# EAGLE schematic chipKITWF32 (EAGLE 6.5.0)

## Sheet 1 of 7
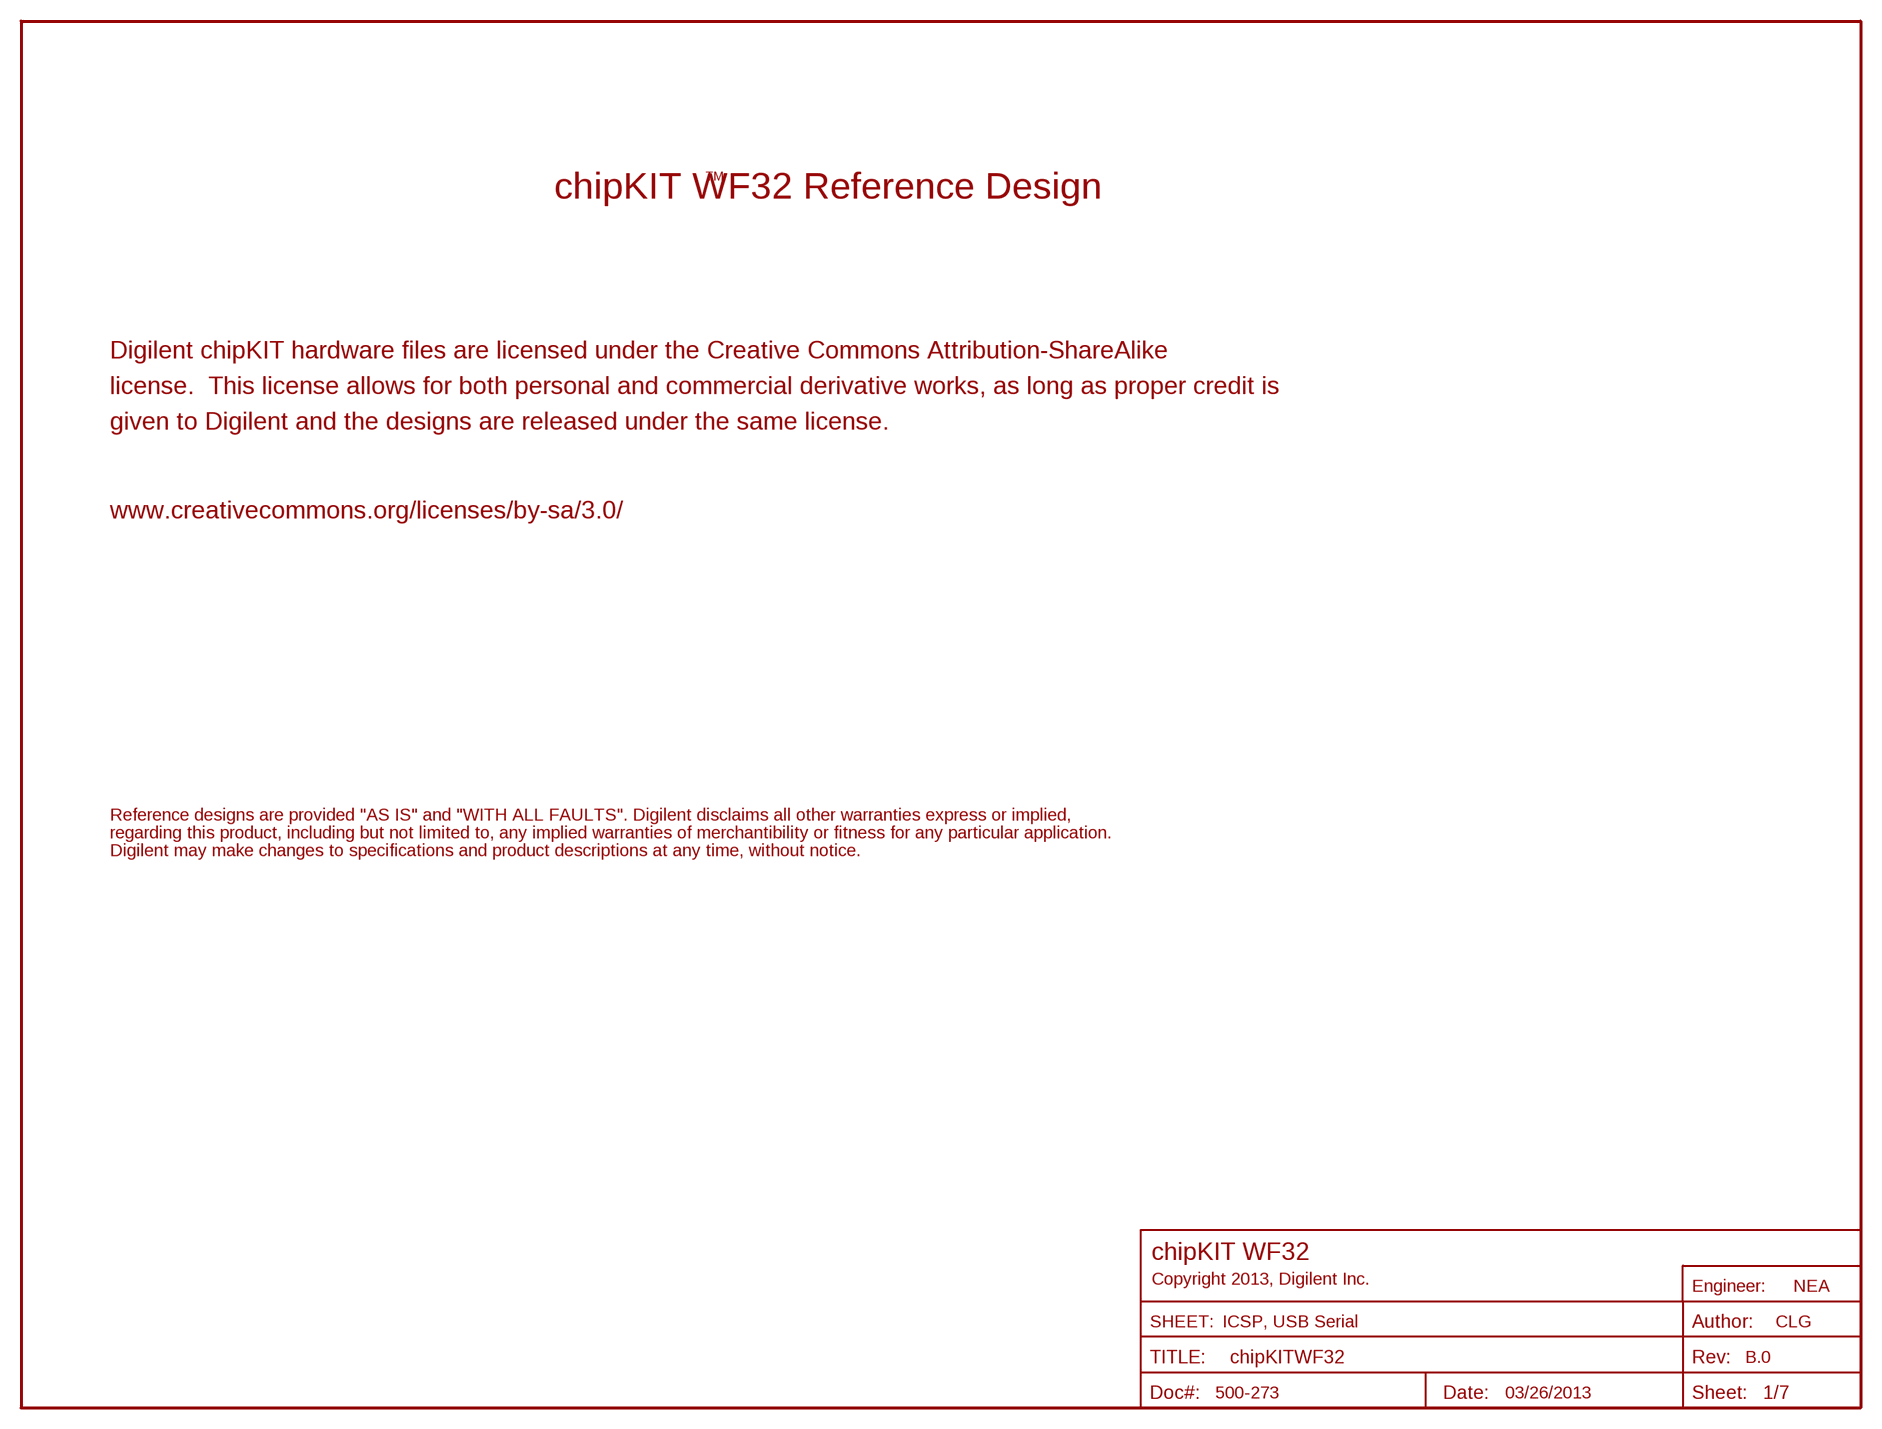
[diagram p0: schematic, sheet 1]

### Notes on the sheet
- TM
- chipKIT WF32 Reference Design
- Digilent chipKIT hardware files are licensed under the Creative Commons Attribution-ShareAlike
- license.  This license allows for both personal and commercial derivative works, as long as proper credit is
- given to Digilent and the designs are released under the same license.
- www.creativecommons.org/licenses/by-sa/3.0/
- Reference designs are provided "AS IS" and "WITH ALL FAULTS". Digilent disclaims all other warranties express or implied,
- regarding this product, including but not limited to, any implied warranties of merchantibility or fitness for any particular application.
- Digilent may make changes to specifications and product descriptions at any time, without notice.
- chipKIT WF32
- Copyright 2013, Digilent Inc.
- NEA
- ICSP, USB Serial | CLG
- B.0
- 500-273 | 03/26/2013

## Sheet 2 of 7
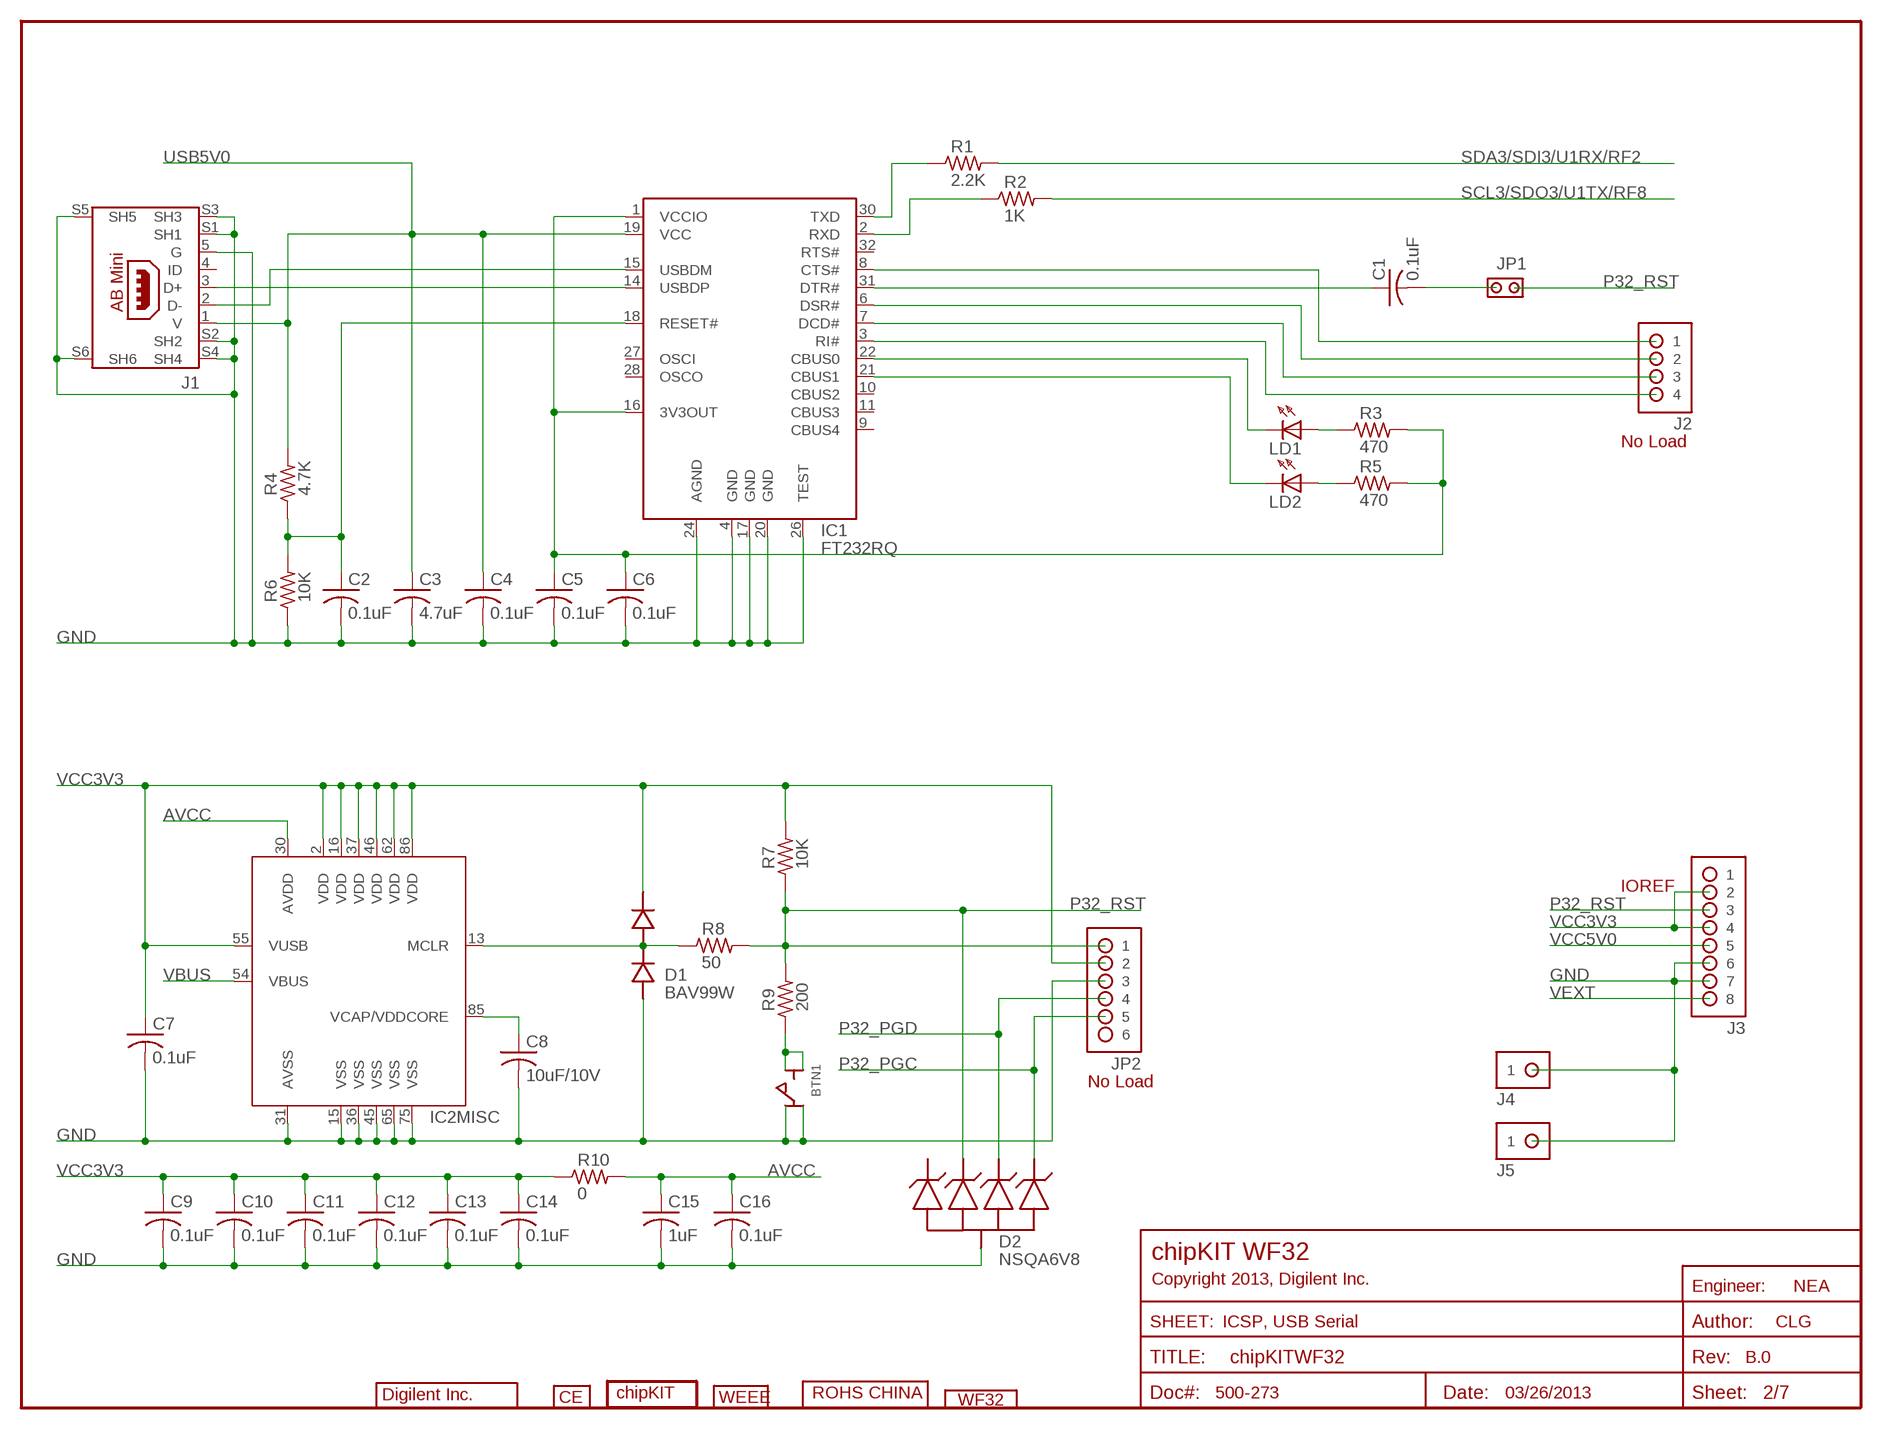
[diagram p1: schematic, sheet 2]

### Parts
BTN1  SW-P8008  [SW-P8008]
C1  0.1uF  CAP-S0402S  [C0402S]
C2  0.1uF  CAP-S0402S  [C0402S]
C3  4.7uF  CAP-S0603S  [C0603S]
C4  0.1uF  CAP-S0402S  [C0402S]
C5  0.1uF  CAP-S0402S  [C0402S]
C6  0.1uF  CAP-S0402S  [C0402S]
C7  0.1uF  CAP-S0402S  [C0402S]
C8  10uF/10V  CAP-S0805S  [C0805S]
C9  0.1uF  CAP-S0402S  [C0402S]
C10  0.1uF  CAP-S0402S  [C0402S]
C11  0.1uF  CAP-S0402S  [C0402S]
C12  0.1uF  CAP-S0402S  [C0402S]
C13  0.1uF  CAP-S0402S  [C0402S]
C14  0.1uF  CAP-S0402S  [C0402S]
C15  1uF  CAP-S0402S  [C0402S]
C16  0.1uF  CAP-S0402S  [C0402S]
D1  BAV99W  [SOT-323]
D2  NSQA6V8  [SOT-323-5]
IC1  FT232RQ  [QFN32]
IC2  PIC32MX695F512L-80I/PT  PIC32MX7X5FL-PT  [TQ100-PT]
J1  USB-AB-MINI  [USB-AB-MINI]
J2  No Load  HDR-1X4  [HDR-1X4]
J3  ST. Female  HDR-1X8  [HDR-1X8]
J4  ST. Male  HDR-1X1  [HDR-1X1]
J5  ST. Male  HDR-1X1  [HDR-1X1]
JP1  ST. Male  JPR-1X2  [JPR-1X2]
JP2  No Load  HDR-1X6-OFFSET  [HDR-1X6_OFFSET]
LD1  Red  LED-S0603S  [D0603S]
LD2  Red  LED-S0603S  [D0603S]
LOGO1  DIGILENT_INC-BT-1000  [DIGILENT_BEYOND_1000_LOGO]
LOGO2  CE  [CE_LOGO]
LOGO3  CHIPKIT  [CHIPKIT_LOGO]
LOGO4  WEEE-S  [WEEE_LOGO]
LOGO5  ROHS-CHINA  [ROHS_CHINA_LOGO]
R1  2.2K  RES-S0402S  [R0402S]
R2  1K  RES-S0402S  [R0402S]
R3  470  RES-S0402S  [R0402S]
R4  4.7K  RES-S0402S  [R0402S]
R5  470  RES-S0402S  [R0402S]
R6  10K  RES-S0402S  [R0402S]
R7  10K  RES-S0402S  [R0402S]
R8  50  RES-S0402S  [R0402S]
R9  200  RES-S0402S  [R0402S]
R10  0  RES-S0603S  [R0603S]
U$1  CHIPKIT_WF32_LOGO  [CHIPKIT_WF32_LOGO]

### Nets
AVCC: C15.1 C16.1 IC2.30(MISC:AVDD) R10.2
FT3V3: C5.1 C6.1 IC1.1(VCCIO) IC1.16(3V3OUT) R3.2 R5.2
GND: BTN1.1A BTN1.2A C2.2 C3.2 C4.2 C5.2 C6.2 C7.2 C8.2 C9.2 C10.2 C11.2 C12.2 C13.2 C14.2 C15.2 C16.2 D1.1(CAT) D2.2(COM) IC1.4(GND) IC1.17(GND) IC1.20(GND) IC1.24(AGND) IC1.26(TEST) IC2.15(MISC:VSS) IC2.31(MISC:AVSS) IC2.36(MISC:VSS) IC2.45(MISC:VSS) IC2.65(MISC:VSS) IC2.75(MISC:VSS) J1.5(G) J1.S1(SH1) J1.S2(SH2) J1.S3(SH3) J1.S4(SH4) J1.S5(SH5) J1.S6(SH6) J3.6 J3.7 J4.1 J5.1 JP2.3 R6.1 ; also sheet 3,4,5,6,7
N$14: C1.2 JP1.2
N$21: D1.3(COM) IC2.13(MISC:MCLR) R8.1
N$24: C8.1 IC2.85(MISC:VCAP/VDDCORE)
N$27: BTN1.1B BTN1.2B R9.1
N$33: IC1.15(USBDM) J1.2(D-)
N$37: IC1.14(USBDP) J1.3(D+)
N$41: IC1.30(TXD) R1.1
N$43: IC1.2(RXD) R2.1
N$47: C2.1 IC1.18(RESET#) R4.1 R6.2
N$52: IC1.8(CTS#) J2.1
N$53: C1.1 IC1.31(DTR#)
N$54: IC1.6(DSR#) J2.2
N$55: IC1.7(DCD#) J2.3
N$56: IC1.3(RI#) J2.4
N$57: IC1.22(CBUS0) LD1.C
N$58: IC1.21(CBUS1) LD2.C
N$59: LD1.A R3.1
N$60: LD2.A R5.1
P32_PGC: D2.5(D4) JP2.5 ; also sheet 4
P32_PGD: D2.4(D3) JP2.4 ; also sheet 4
P32_RST: D2.3(D2) J3.3 JP1.1 JP2.1 R7.1 R8.2 R9.2
SCL3/SDO3/U1TX/RF8: R2.2 ; also sheet 3,5
SDA3/SDI3/U1RX/RF2: R1.2 ; also sheet 3,5
USB5V0: C3.1 C4.1 IC1.19(VCC) J1.1(V) R4.2 ; also sheet 7
VBUS: IC2.54(MISC:VBUS) ; also sheet 6,7
VCC3V3: C7.1 C9.1 C10.1 C11.1 C12.1 C13.1 C14.1 D1.2(AN) IC2.2(MISC:VDD) IC2.16(MISC:VDD) IC2.37(MISC:VDD) IC2.46(MISC:VDD) IC2.55(MISC:VUSB) IC2.62(MISC:VDD) IC2.86(MISC:VDD) J3.2 J3.4 JP2.2 R7.2 R10.1 ; also sheet 4,6,7
VCC5V0: J3.5 ; also sheet 6,7
VEXT: J3.8 ; also sheet 7
Unconnected: D2.1(D1) IC1.9(CBUS4) IC1.10(CBUS2) IC1.11(CBUS3) IC1.27(OSCI) IC1.28(OSCO) IC1.32(RTS#) J1.4(ID) J3.1 JP2.6

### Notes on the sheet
- No Load
- IOREF
- No Load
- chipKIT WF32
- Copyright 2013, Digilent Inc.
- NEA
- ICSP, USB Serial | CLG
- B.0
- 500-273 | 03/26/2013

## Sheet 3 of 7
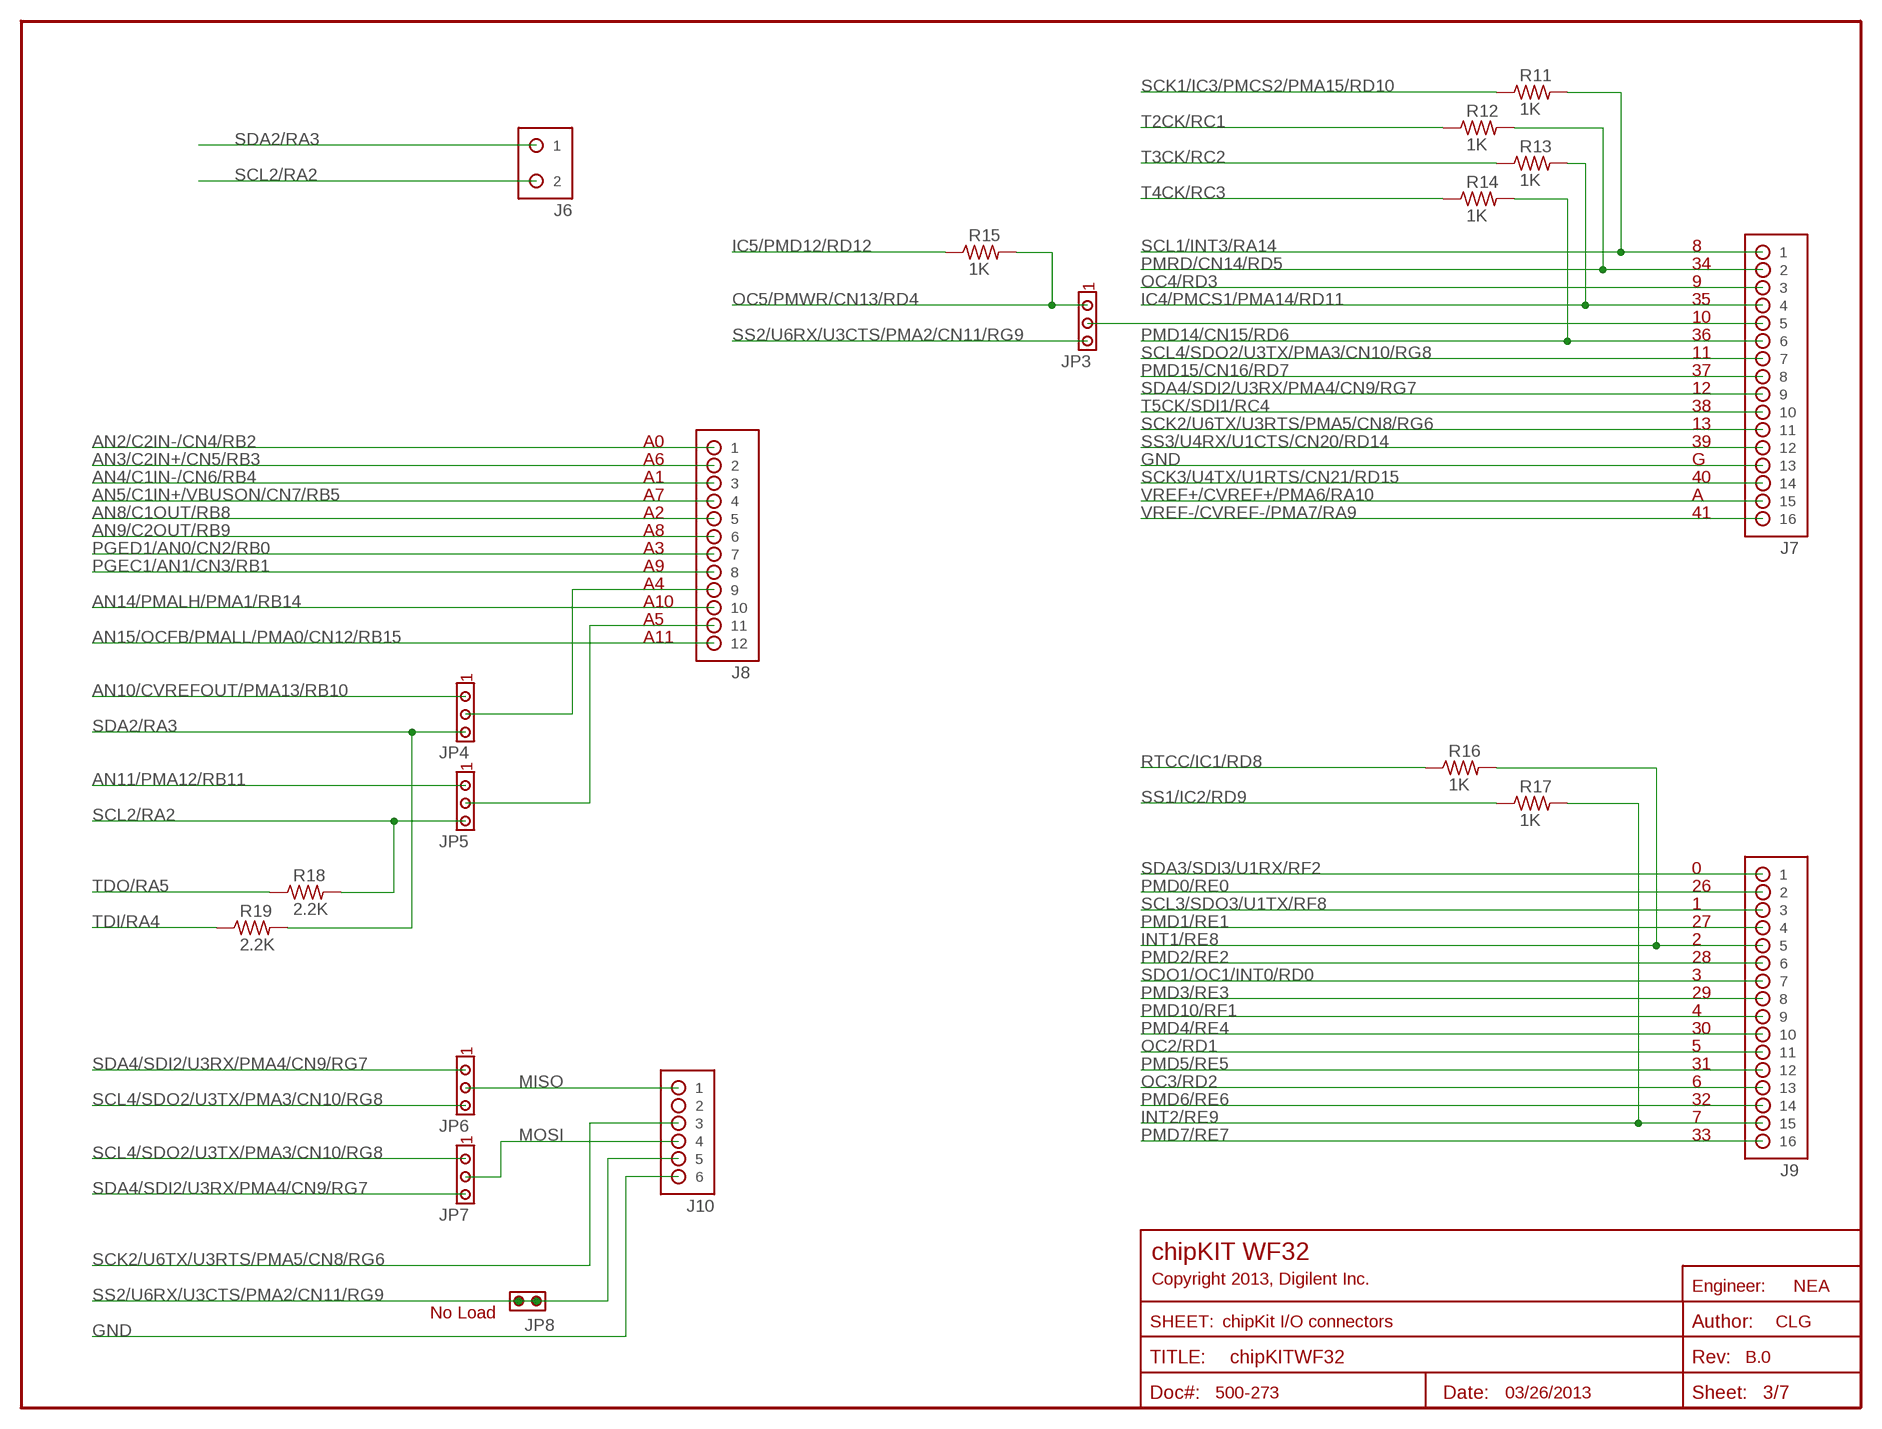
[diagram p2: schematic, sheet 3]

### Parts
J6  ST. Female  HDR-1X2  [HDR-1X2]
J7  ST. Female  HDR-2X8  [HDR-2X8]
J8  ST. Female  HDR-2X6  [HDR-2X6]
J9  ST. Female  HDR-2X8  [HDR-2X8]
J10  ST. Male  HDR-2X3  [HDR-2X3]
JP3  JPR-1X3  [JPR-1X3]
JP4  ST. Male  JPR-1X3  [JPR-1X3]
JP5  ST. Male  JPR-1X3  [JPR-1X3]
JP6  JPR-1X3  [JPR-1X3]
JP7  JPR-1X3  [JPR-1X3]
JP8  No Load  JPR-1X2  [JPR-1X2]
R11  1K  RES-S0402S  [R0402S]
R12  1K  RES-S0402S  [R0402S]
R13  1K  RES-S0402S  [R0402S]
R14  1K  RES-S0402S  [R0402S]
R15  1K  RES-S0402S  [R0402S]
R16  1K  RES-S0402S  [R0402S]
R17  1K  RES-S0402S  [R0402S]
R18  2.2K  RES-S0402S  [R0402S]
R19  2.2K  RES-S0402S  [R0402S]

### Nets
AN2/C2IN-/CN4/RB2: J8.1 ; also sheet 4
AN3/C2IN+/CN5/RB3: J8.2 ; also sheet 4
AN4/C1IN-/CN6/RB4: J8.3 ; also sheet 4
AN5/C1IN+/VBUSON/CN7/RB5: J8.4 ; also sheet 4,6
AN8/C1OUT/RB8: J8.5 ; also sheet 4
AN9/C2OUT/RB9: J8.6 ; also sheet 4
AN10/CVREFOUT/PMA13/RB10: JP4.1 ; also sheet 4
AN11/PMA12/RB11: JP5.1 ; also sheet 4
AN14/PMALH/PMA1/RB14: J8.10 ; also sheet 4
AN15/OCFB/PMALL/PMA0/CN12/RB15: J8.12 ; also sheet 4
GND: J7.13 J10.6 ; also sheet 2,4,5,6,7
IC4/PMCS1/PMA14/RD11: J7.4 R13.2 ; also sheet 5
IC5/PMD12/RD12: R15.1 ; also sheet 5
INT1/RE8: J9.5 R16.2 ; also sheet 5
INT2/RE9: J9.15 R17.2 ; also sheet 5
MISO: J10.1 JP6.2
MOSI: J10.4 JP7.2
N$46: J8.9 JP4.2
N$49: J8.11 JP5.2
N$50: J7.5 JP3.2
OC2/RD1: J9.11 ; also sheet 5
OC3/RD2: J9.13 ; also sheet 5
OC4/RD3: J7.3 ; also sheet 5
OC5/PMWR/CN13/RD4: JP3.1 R15.2 ; also sheet 5
PGEC1/AN1/CN3/RB1: J8.8 ; also sheet 4
PGED1/AN0/CN2/RB0: J8.7 ; also sheet 4
PMD0/RE0: J9.2 ; also sheet 5
PMD1/RE1: J9.4 ; also sheet 5
PMD2/RE2: J9.6 ; also sheet 5
PMD3/RE3: J9.8 ; also sheet 5
PMD4/RE4: J9.10 ; also sheet 5
PMD5/RE5: J9.12 ; also sheet 5
PMD6/RE6: J9.14 ; also sheet 5
PMD7/RE7: J9.16 ; also sheet 5
PMD10/RF1: J9.9 ; also sheet 5
PMD14/CN15/RD6: J7.6 R14.2 ; also sheet 5
PMD15/CN16/RD7: J7.8 ; also sheet 5
PMRD/CN14/RD5: J7.2 R12.2 ; also sheet 5
RTCC/IC1/RD8: R16.1 ; also sheet 5
SCK1/IC3/PMCS2/PMA15/RD10: R11.1 ; also sheet 5
SCK2/U6TX/U3RTS/PMA5/CN8/RG6: J7.11 J10.3 ; also sheet 5,6
SCK3/U4TX/U1RTS/CN21/RD15: J7.14 ; also sheet 5
SCL1/INT3/RA14: J7.1 R11.2 ; also sheet 4,6
SCL2/RA2: J6.2 JP5.3 R18.2 ; also sheet 4
SCL3/SDO3/U1TX/RF8: J9.3 ; also sheet 2,5
SCL4/SDO2/U3TX/PMA3/CN10/RG8: J7.7 JP6.3 JP7.1 ; also sheet 5
SDA2/RA3: J6.1 JP4.3 R19.2 ; also sheet 4
SDA3/SDI3/U1RX/RF2: J9.1 ; also sheet 2,5
SDA4/SDI2/U3RX/PMA4/CN9/RG7: J7.9 JP6.1 JP7.3 ; also sheet 5
SDO1/OC1/INT0/RD0: J9.7 ; also sheet 5
SS1/IC2/RD9: R17.1 ; also sheet 5
SS2/U6RX/U3CTS/PMA2/CN11/RG9: J10.5 JP3.3 JP8.1 JP8.2 ; also sheet 5
SS3/U4RX/U1CTS/CN20/RD14: J7.12 ; also sheet 5
T2CK/RC1: R12.1 ; also sheet 5
T3CK/RC2: R13.1 ; also sheet 5
T4CK/RC3: R14.1 ; also sheet 5
T5CK/SDI1/RC4: J7.10 ; also sheet 5
TDI/RA4: R19.1 ; also sheet 4
TDO/RA5: R18.1 ; also sheet 4
VREF+/CVREF+/PMA6/RA10: J7.15 ; also sheet 4
VREF-/CVREF-/PMA7/RA9: J7.16 ; also sheet 4
Unconnected: J10.2

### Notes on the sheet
- 8
- 34
- 9
- 35
- 10
- 36
- 11
- 37
- 12
- 38
- 13
- A0 | 39
- A6 | G
- A1 | 40
- A7 | A
- A2 | 41
- A8
- A3
- A9
- A4
- A10
- A5
- A11
- 0
- 26
- 1
- 27
- 2
- 28
- 3
- 29
- 4
- 30
- 5
- 31
- 6
- 32
- 7
- 33
- chipKIT WF32
- Copyright 2013, Digilent Inc.
- NEA
- No Load
- chipKit I/O connectors | CLG
- B.0
- 500-273 | 03/26/2013

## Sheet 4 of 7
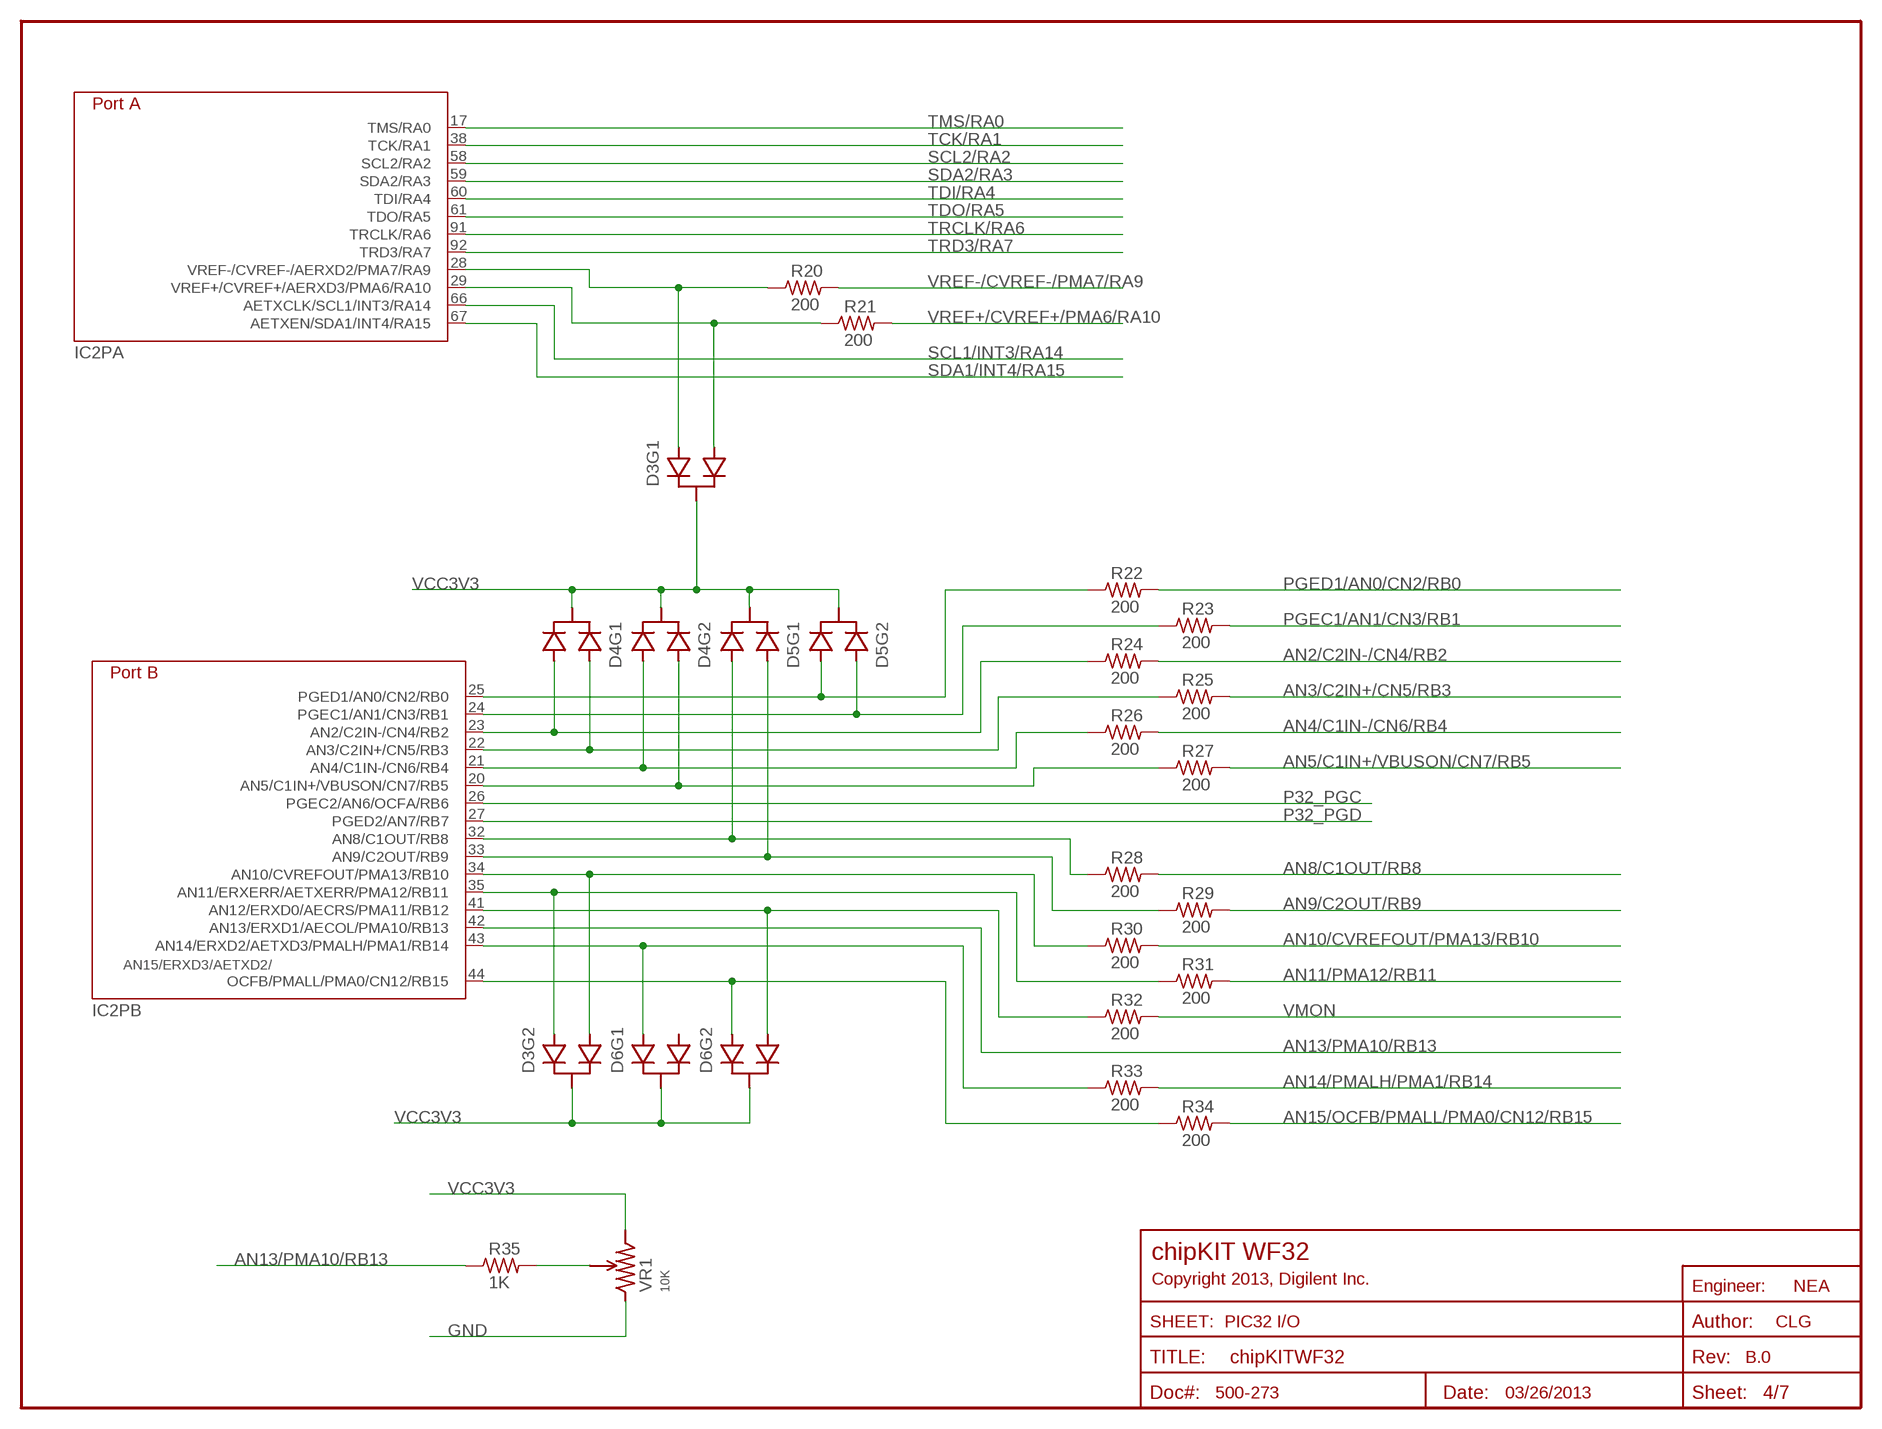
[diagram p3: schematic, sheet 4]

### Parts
D3  BAV70S  [SOT-363]
D4  BAV70S  [SOT-363]
D5  BAV70S  [SOT-363]
D6  BAV70S  [SOT-363]
R20  200  RES-S0402S  [R0402S]
R21  200  RES-S0402S  [R0402S]
R22  200  RES-S0402S  [R0402S]
R23  200  RES-S0402S  [R0402S]
R24  200  RES-S0402S  [R0402S]
R25  200  RES-S0402S  [R0402S]
R26  200  RES-S0402S  [R0402S]
R27  200  RES-S0402S  [R0402S]
R28  200  RES-S0402S  [R0402S]
R29  200  RES-S0402S  [R0402S]
R30  200  RES-S0402S  [R0402S]
R31  200  RES-S0402S  [R0402S]
R32  200  RES-S0402S  [R0402S]
R33  200  RES-S0402S  [R0402S]
R34  200  RES-S0402S  [R0402S]
R35  1K  RES-S0402S  [R0402S]
VR1  10K  POT-3352T  [BOURNS-3352T]

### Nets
AN2/C2IN-/CN4/RB2: R24.2 ; also sheet 3
AN3/C2IN+/CN5/RB3: R25.2 ; also sheet 3
AN4/C1IN-/CN6/RB4: R26.2 ; also sheet 3
AN5/C1IN+/VBUSON/CN7/RB5: R27.2 ; also sheet 3,6
AN8/C1OUT/RB8: R28.2 ; also sheet 3
AN9/C2OUT/RB9: R29.2 ; also sheet 3
AN10/CVREFOUT/PMA13/RB10: R30.2 ; also sheet 3
AN11/PMA12/RB11: R31.2 ; also sheet 3
AN13/PMA10/RB13: IC2.42(PB:AN13/ERXD1/AECOL/PMA10/RB13) R35.1
AN14/PMALH/PMA1/RB14: R33.2 ; also sheet 3
AN15/OCFB/PMALL/PMA0/CN12/RB15: R34.2 ; also sheet 3
GND: VR1.1 ; also sheet 2,3,5,6,7
N$1: D5.4(A1) IC2.25(PB:PGED1/AN0/CN2/RB0) R22.1
N$2: D5.5(A2) IC2.24(PB:PGEC1/AN1/CN3/RB1) R23.1
N$3: D4.1(A1) IC2.23(PB:AN2/C2IN-/CN4/RB2) R24.1
N$4: D4.2(A2) IC2.22(PB:AN3/C2IN+/CN5/RB3) R25.1
N$5: D4.4(A1) IC2.21(PB:AN4/C1IN-/CN6/RB4) R26.1
N$6: D4.5(A2) IC2.20(PB:AN5/C1IN+/VBUSON/CN7/RB5) R27.1
N$9: D5.1(A1) IC2.32(PB:AN8/C1OUT/RB8) R28.1
N$10: D5.2(A2) IC2.33(PB:AN9/C2OUT/RB9) R29.1
N$11: D3.4(A1) IC2.34(PB:AN10/CVREFOUT/PMA13/RB10) R30.1
N$12: D3.5(A2) IC2.35(PB:AN11/ERXERR/AETXERR/PMA12/RB11) R31.1
N$13: D6.4(A1) IC2.41(PB:AN12/ERXD0/AECRS/PMA11/RB12) R32.1
N$15: D6.2(A2) IC2.43(PB:AN14/ERXD2/AETXD3/PMALH/PMA1/RB14) R33.1
N$16: D6.5(A2) IC2.44(PB:OCFB/PMALL/PMA0/CN12/RB15) R34.1
N$40: R35.2 VR1.2
N$48: D3.2(A2) IC2.28(PA:VREF-/CVREF-/AERXD2/PMA7/RA9) R20.1
N$61: D3.1(A1) IC2.29(PA:VREF+/CVREF+/AERXD3/PMA6/RA10) R21.1
P32_PGC: IC2.26(PB:PGEC2/AN6/OCFA/RB6) ; also sheet 2
P32_PGD: IC2.27(PB:PGED2/AN7/RB7) ; also sheet 2
PGEC1/AN1/CN3/RB1: R23.2 ; also sheet 3
PGED1/AN0/CN2/RB0: R22.2 ; also sheet 3
SCL1/INT3/RA14: IC2.66(PA:AETXCLK/SCL1/INT3/RA14) ; also sheet 3,6
SCL2/RA2: IC2.58(PA:SCL2/RA2) ; also sheet 3
SDA1/INT4/RA15: IC2.67(PA:AETXEN/SDA1/INT4/RA15) ; also sheet 6
SDA2/RA3: IC2.59(PA:SDA2/RA3) ; also sheet 3
TCK/RA1: IC2.38(PA:TCK/RA1) ; also sheet 6
TDI/RA4: IC2.60(PA:TDI/RA4) ; also sheet 3
TDO/RA5: IC2.61(PA:TDO/RA5) ; also sheet 3
TMS/RA0: IC2.17(PA:TMS/RA0) ; also sheet 6
TRCLK/RA6: IC2.91(PA:TRCLK/RA6) ; also sheet 6
TRD3/RA7: IC2.92(PA:TRD3/RA7) ; also sheet 6
VCC3V3: D3.3(K) D3.6(K) D4.3(K) D4.6(K) D5.3(K) D5.6(K) D6.3(K) D6.6(K) VR1.3 ; also sheet 2,6,7
VMON: R32.2 ; also sheet 7
VREF+/CVREF+/PMA6/RA10: R21.2 ; also sheet 3
VREF-/CVREF-/PMA7/RA9: R20.2 ; also sheet 3
Unconnected: D6.1(A1)

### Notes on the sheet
- chipKIT WF32
- Copyright 2013, Digilent Inc.
- NEA
- PIC32 I/O | CLG
- B.0
- 500-273 | 03/26/2013

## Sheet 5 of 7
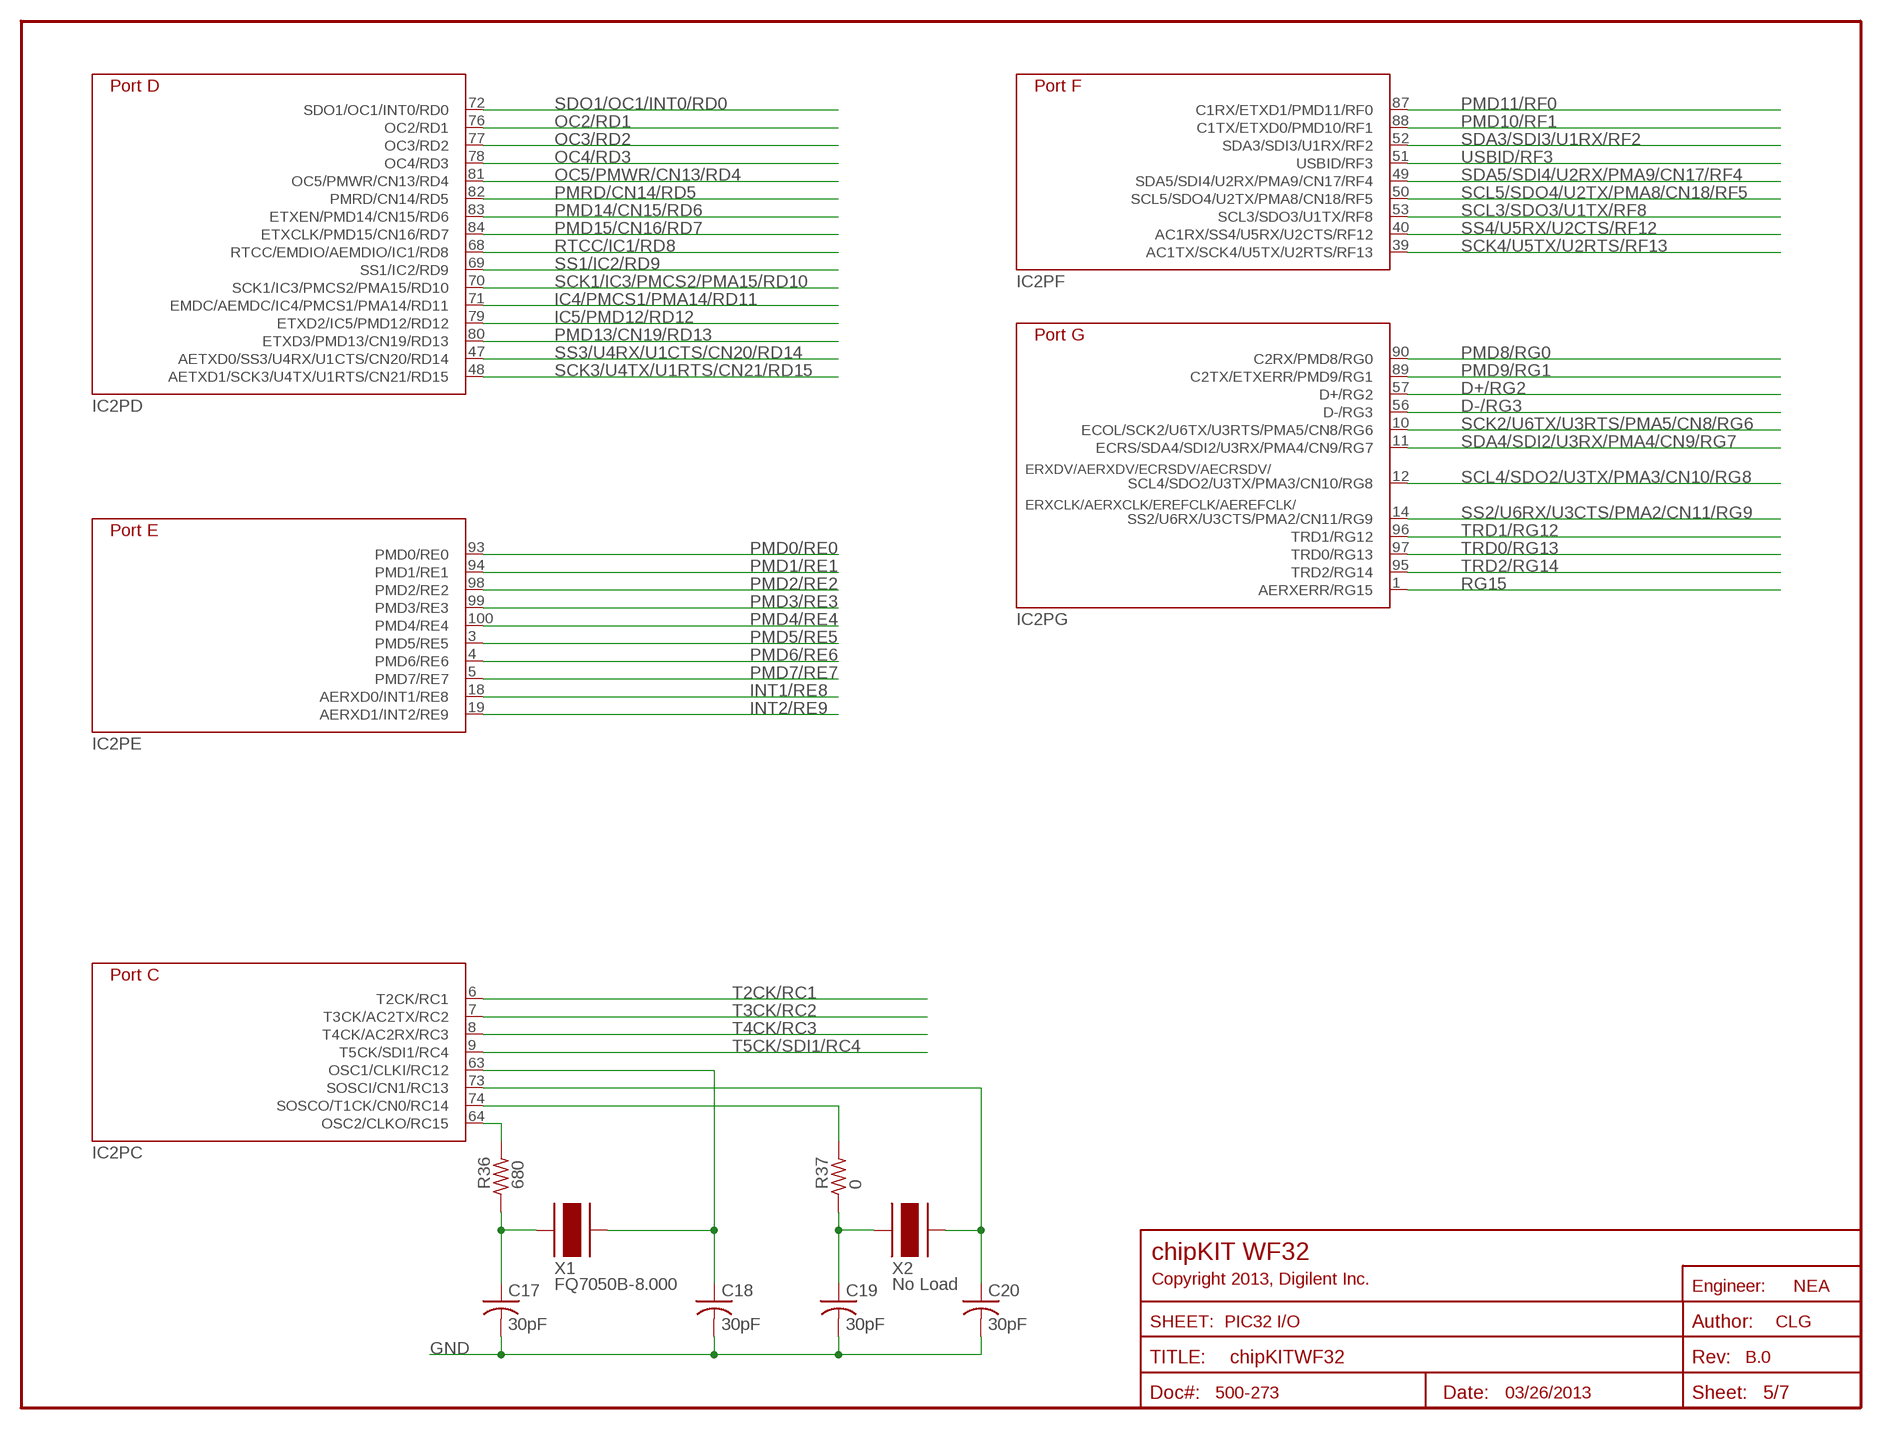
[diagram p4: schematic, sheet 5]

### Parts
C17  30pF  CAP-S0402S  [C0402S]
C18  30pF  CAP-S0402S  [C0402S]
C19  30pF  CAP-S0402S  [C0402S]
C20  30pF  CAP-S0402S  [C0402S]
R36  680  RES-S0402S  [R0402S]
R37  0  RES-S0402S  [R0402S]
X1  FQ7050B-8.000  XTAL-FQ7050B  [FQ7050B]
X2  No Load  XTAL-T38  [XT-T38]

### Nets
D+/RG2: IC2.57(PG:D+/RG2) ; also sheet 6
D-/RG3: IC2.56(PG:D-/RG3) ; also sheet 6
GND: C17.2 C18.2 C19.2 C20.2 ; also sheet 2,3,4,6,7
IC4/PMCS1/PMA14/RD11: IC2.71(PD:EMDC/AEMDC/IC4/PMCS1/PMA14/RD11) ; also sheet 3
IC5/PMD12/RD12: IC2.79(PD:ETXD2/IC5/PMD12/RD12) ; also sheet 3
INT1/RE8: IC2.18(PE:AERXD0/INT1/RE8) ; also sheet 3
INT2/RE9: IC2.19(PE:AERXD1/INT2/RE9) ; also sheet 3
N$7: IC2.64(PC:OSC2/CLKO/RC15) R36.2
N$8: C17.1 R36.1 X1.1
N$17: C18.1 IC2.63(PC:OSC1/CLKI/RC12) X1.3
N$18: C20.1 IC2.73(PC:SOSCI/CN1/RC13) X2.2
N$19: IC2.74(PC:SOSCO/T1CK/CN0/RC14) R37.2
N$20: C19.1 R37.1 X2.1
OC2/RD1: IC2.76(PD:OC2/RD1) ; also sheet 3
OC3/RD2: IC2.77(PD:OC3/RD2) ; also sheet 3
OC4/RD3: IC2.78(PD:OC4/RD3) ; also sheet 3
OC5/PMWR/CN13/RD4: IC2.81(PD:OC5/PMWR/CN13/RD4) ; also sheet 3
PMD0/RE0: IC2.93(PE:PMD0/RE0) ; also sheet 3
PMD1/RE1: IC2.94(PE:PMD1/RE1) ; also sheet 3
PMD2/RE2: IC2.98(PE:PMD2/RE2) ; also sheet 3
PMD3/RE3: IC2.99(PE:PMD3/RE3) ; also sheet 3
PMD4/RE4: IC2.100(PE:PMD4/RE4) ; also sheet 3
PMD5/RE5: IC2.3(PE:PMD5/RE5) ; also sheet 3
PMD6/RE6: IC2.4(PE:PMD6/RE6) ; also sheet 3
PMD7/RE7: IC2.5(PE:PMD7/RE7) ; also sheet 3
PMD8/RG0: IC2.90(PG:C2RX/PMD8/RG0) ; also sheet 6
PMD9/RG1: IC2.89(PG:C2TX/ETXERR/PMD9/RG1) ; also sheet 6
PMD10/RF1: IC2.88(PF:C1TX/ETXD0/PMD10/RF1) ; also sheet 3
PMD11/RF0: IC2.87(PF:C1RX/ETXD1/PMD11/RF0) ; also sheet 6
PMD13/CN19/RD13: IC2.80(PD:ETXD3/PMD13/CN19/RD13) ; also sheet 7
PMD14/CN15/RD6: IC2.83(PD:ETXEN/PMD14/CN15/RD6) ; also sheet 3
PMD15/CN16/RD7: IC2.84(PD:ETXCLK/PMD15/CN16/RD7) ; also sheet 3
PMRD/CN14/RD5: IC2.82(PD:PMRD/CN14/RD5) ; also sheet 3
RG15: IC2.1(PG:AERXERR/RG15) ; also sheet 6
RTCC/IC1/RD8: IC2.68(PD:RTCC/EMDIO/AEMDIO/IC1/RD8) ; also sheet 3
SCK1/IC3/PMCS2/PMA15/RD10: IC2.70(PD:SCK1/IC3/PMCS2/PMA15/RD10) ; also sheet 3
SCK2/U6TX/U3RTS/PMA5/CN8/RG6: IC2.10(PG:ECOL/SCK2/U6TX/U3RTS/PMA5/CN8/RG6) ; also sheet 3,6
SCK3/U4TX/U1RTS/CN21/RD15: IC2.48(PD:AETXD1/SCK3/U4TX/U1RTS/CN21/RD15) ; also sheet 3
SCK4/U5TX/U2RTS/RF13: IC2.39(PF:AC1TX/SCK4/U5TX/U2RTS/RF13) ; also sheet 6
SCL3/SDO3/U1TX/RF8: IC2.53(PF:SCL3/SDO3/U1TX/RF8) ; also sheet 2,3
SCL4/SDO2/U3TX/PMA3/CN10/RG8: IC2.12(PG:SCL4/SDO2/U3TX/PMA3/CN10/RG8) ; also sheet 3
SCL5/SDO4/U2TX/PMA8/CN18/RF5: IC2.50(PF:SCL5/SDO4/U2TX/PMA8/CN18/RF5) ; also sheet 6
SDA3/SDI3/U1RX/RF2: IC2.52(PF:SDA3/SDI3/U1RX/RF2) ; also sheet 2,3
SDA4/SDI2/U3RX/PMA4/CN9/RG7: IC2.11(PG:ECRS/SDA4/SDI2/U3RX/PMA4/CN9/RG7) ; also sheet 3
SDA5/SDI4/U2RX/PMA9/CN17/RF4: IC2.49(PF:SDA5/SDI4/U2RX/PMA9/CN17/RF4) ; also sheet 6
SDO1/OC1/INT0/RD0: IC2.72(PD:SDO1/OC1/INT0/RD0) ; also sheet 3
SS1/IC2/RD9: IC2.69(PD:SS1/IC2/RD9) ; also sheet 3
SS2/U6RX/U3CTS/PMA2/CN11/RG9: IC2.14(PG:SS2/U6RX/U3CTS/PMA2/CN11/RG9) ; also sheet 3
SS3/U4RX/U1CTS/CN20/RD14: IC2.47(PD:AETXD0/SS3/U4RX/U1CTS/CN20/RD14) ; also sheet 3
SS4/U5RX/U2CTS/RF12: IC2.40(PF:AC1RX/SS4/U5RX/U2CTS/RF12) ; also sheet 6
T2CK/RC1: IC2.6(PC:T2CK/RC1) ; also sheet 3
T3CK/RC2: IC2.7(PC:T3CK/AC2TX/RC2) ; also sheet 3
T4CK/RC3: IC2.8(PC:T4CK/AC2RX/RC3) ; also sheet 3
T5CK/SDI1/RC4: IC2.9(PC:T5CK/SDI1/RC4) ; also sheet 3
TRD0/RG13: IC2.97(PG:TRD0/RG13) ; also sheet 6
TRD1/RG12: IC2.96(PG:TRD1/RG12) ; also sheet 6
TRD2/RG14: IC2.95(PG:TRD2/RG14) ; also sheet 6
USBID/RF3: IC2.51(PF:USBID/RF3) ; also sheet 6

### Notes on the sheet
- chipKIT WF32
- Copyright 2013, Digilent Inc.
- NEA
- PIC32 I/O | CLG
- B.0
- 500-273 | 03/26/2013

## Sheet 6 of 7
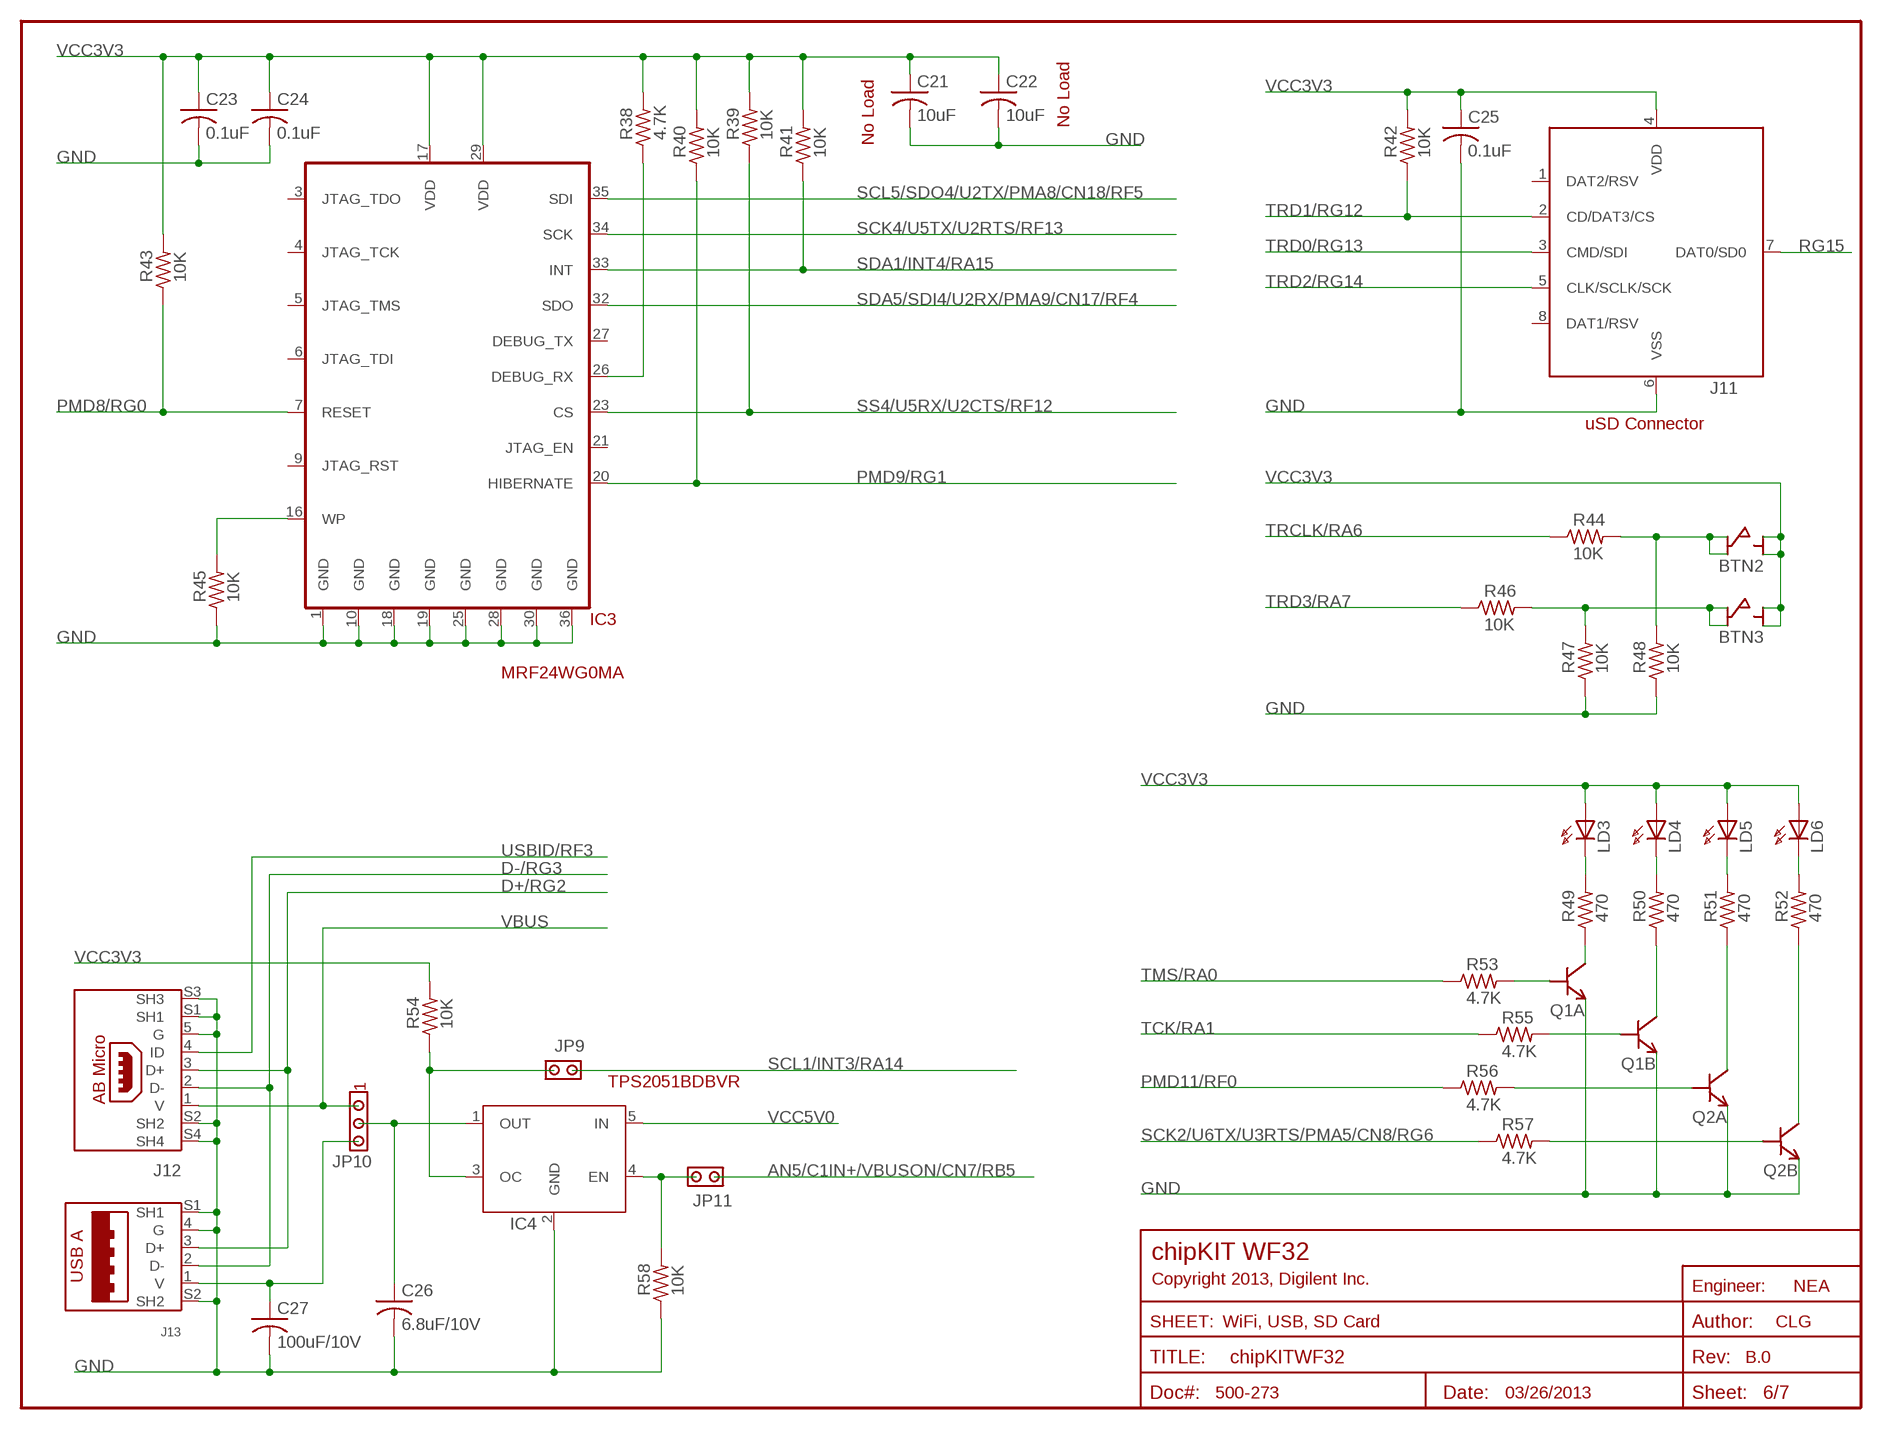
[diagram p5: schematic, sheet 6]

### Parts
BTN2  SW-P8008  [SW-P8008]
BTN3  SW-P8008  [SW-P8008]
C21  10uF  CAP-S0805S  [C0805S]
C22  10uF  CAP-S0805S  [C0805S]
C23  0.1uF  CAP-S0402S  [C0402S]
C24  0.1uF  CAP-S0402S  [C0402S]
C25  0.1uF  CAP-S0402S  [C0402S]
C26  6.8uF/10V  CAP-S0603S  [C0603S]
C27  100uF/10V  CAP-S1206S  [C1206S]
IC3  MRF24WG0MA  MRF24WB0MA  [MRF24WB0MA]
IC4  TPS2051BDBVR  TPS2041B-DBV  [SOT23-5]
J11  2908-05WB-MG  [2908-05WB-MG]
J12  USB-AB-MICRO  [USB-AB-MICRO]
J13  USB-A  [USB-A]
JP9  ST. Male  JPR-1X2  [JPR-1X2]
JP10  ST. Male  JPR-1X3  [JPR-1X3]
JP11  ST. Male  JPR-1X2  [JPR-1X2]
LD3  Green  LED-S0603S  [D0603S]
LD4  Green  LED-S0603S  [D0603S]
LD5  Green  LED-S0603S  [D0603S]
LD6  Green  LED-S0603S  [D0603S]
Q1  MBT3904DW1T1  [SOT-363]
Q2  MBT3904DW1T1  [SOT-363]
R38  4.7K  RES-S0402S  [R0402S]
R39  10K  RES-S0402S  [R0402S]
R40  10K  RES-S0402S  [R0402S]
R41  10K  RES-S0402S  [R0402S]
R42  10K  RES-S0402S  [R0402S]
R43  10K  RES-S0402S  [R0402S]
R44  10K  RES-S0402S  [R0402S]
R45  10K  RES-S0402S  [R0402S]
R46  10K  RES-S0402S  [R0402S]
R47  10K  RES-S0402S  [R0402S]
R48  10K  RES-S0402S  [R0402S]
R49  470  RES-S0402S  [R0402S]
R50  470  RES-S0402S  [R0402S]
R51  470  RES-S0402S  [R0402S]
R52  470  RES-S0402S  [R0402S]
R53  4.7K  RES-S0402S  [R0402S]
R54  10K  RES-S0402S  [R0402S]
R55  4.7K  RES-S0402S  [R0402S]
R56  4.7K  RES-S0402S  [R0402S]
R57  4.7K  RES-S0402S  [R0402S]
R58  10K  RES-S0402S  [R0402S]

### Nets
AN5/C1IN+/VBUSON/CN7/RB5: JP11.2 ; also sheet 3,4
D+/RG2: J12.3(D+) J13.3(D+) ; also sheet 5
D-/RG3: J12.2(D-) J13.2(D-) ; also sheet 5
GND: C21.2 C22.2 C23.2 C24.2 C25.2 C26.2 C27.2 IC3.1(GND) IC3.10(GND) IC3.18(GND) IC3.19(GND) IC3.25(GND) IC3.28(GND) IC3.30(GND) IC3.36(GND) IC4.2(GND) J11.6(VSS) J12.5(G) J12.S1(SH1) J12.S2(SH2) J12.S3(SH3) J12.S4(SH4) J13.4(G) J13.S1(SH1) J13.S2(SH2) Q1.1(B:E) Q1.4(A:E) Q2.1(B:E) Q2.4(A:E) R45.1 R47.1 R48.1 R58.1 ; also sheet 2,3,4,5,7
N$22: Q2.5(A:B) R56.2
N$23: Q2.3(A:C) R51.1
N$25: IC4.3(OC) JP9.1 R54.1
N$26: LD5.C R51.2
N$28: LD6.C R52.2
N$29: IC3.26(DEBUG_RX) R38.1
N$31: Q2.2(B:B) R57.2
N$32: Q2.6(B:C) R52.1
N$45: IC3.16(WP) R45.2
N$51: LD4.C R50.2
N$62: IC4.4(EN) JP11.1 R58.2
N$63: LD3.C R49.2
N$64: Q1.6(B:C) R50.1
N$65: Q1.3(A:C) R49.1
N$66: C27.1 J13.1(V) JP10.3
N$67: Q1.2(B:B) R55.2
N$68: C26.1 IC4.1(OUT) JP10.2
N$69: Q1.5(A:B) R53.2
N$71: BTN2.1A BTN2.2A R44.2 R48.2
N$72: BTN3.1A BTN3.2A R46.2 R47.2
PMD8/RG0: IC3.7(RESET) R43.1 ; also sheet 5
PMD9/RG1: IC3.20(HIBERNATE) R40.1 ; also sheet 5
PMD11/RF0: R56.1 ; also sheet 5
RG15: J11.7(DAT0/SD0) ; also sheet 5
SCK2/U6TX/U3RTS/PMA5/CN8/RG6: R57.1 ; also sheet 3,5
SCK4/U5TX/U2RTS/RF13: IC3.34(SCK) ; also sheet 5
SCL1/INT3/RA14: JP9.2 ; also sheet 3,4
SCL5/SDO4/U2TX/PMA8/CN18/RF5: IC3.35(SDI) ; also sheet 5
SDA1/INT4/RA15: IC3.33(INT) R41.1 ; also sheet 4
SDA5/SDI4/U2RX/PMA9/CN17/RF4: IC3.32(SDO) ; also sheet 5
SS4/U5RX/U2CTS/RF12: IC3.23(CS) R39.1 ; also sheet 5
TCK/RA1: R55.1 ; also sheet 4
TMS/RA0: R53.1 ; also sheet 4
TRCLK/RA6: R44.1 ; also sheet 4
TRD0/RG13: J11.3(CMD/SDI) ; also sheet 5
TRD1/RG12: J11.2(CD/DAT3/CS) R42.1 ; also sheet 5
TRD2/RG14: J11.5(CLK/SCLK/SCK) ; also sheet 5
TRD3/RA7: R46.1 ; also sheet 4
USBID/RF3: J12.4(ID) ; also sheet 5
VBUS: J12.1(V) JP10.1 ; also sheet 2,7
VCC3V3: BTN2.1B BTN2.2B BTN3.1B BTN3.2B C21.1 C22.1 C23.1 C24.1 C25.1 IC3.17(VDD) IC3.29(VDD) J11.4(VDD) LD3.A LD4.A LD5.A LD6.A R38.2 R39.2 R40.2 R41.2 R42.2 R43.2 R54.2 ; also sheet 2,4,7
VCC5V0: IC4.5(IN) ; also sheet 2,7
Unconnected: IC3.3(JTAG_TDO) IC3.4(JTAG_TCK) IC3.5(JTAG_TMS) IC3.6(JTAG_TDI) IC3.9(JTAG_RST) IC3.21(JTAG_EN) IC3.27(DEBUG_TX) J11.1(DAT2/RSV) J11.8(DAT1/RSV)

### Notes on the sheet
- No Load
- No Load
- uSD Connector
- MRF24WG0MA
- TPS2051BDBVR
- chipKIT WF32
- Copyright 2013, Digilent Inc.
- NEA
- WiFi, USB, SD Card | CLG
- B.0
- 500-273 | 03/26/2013

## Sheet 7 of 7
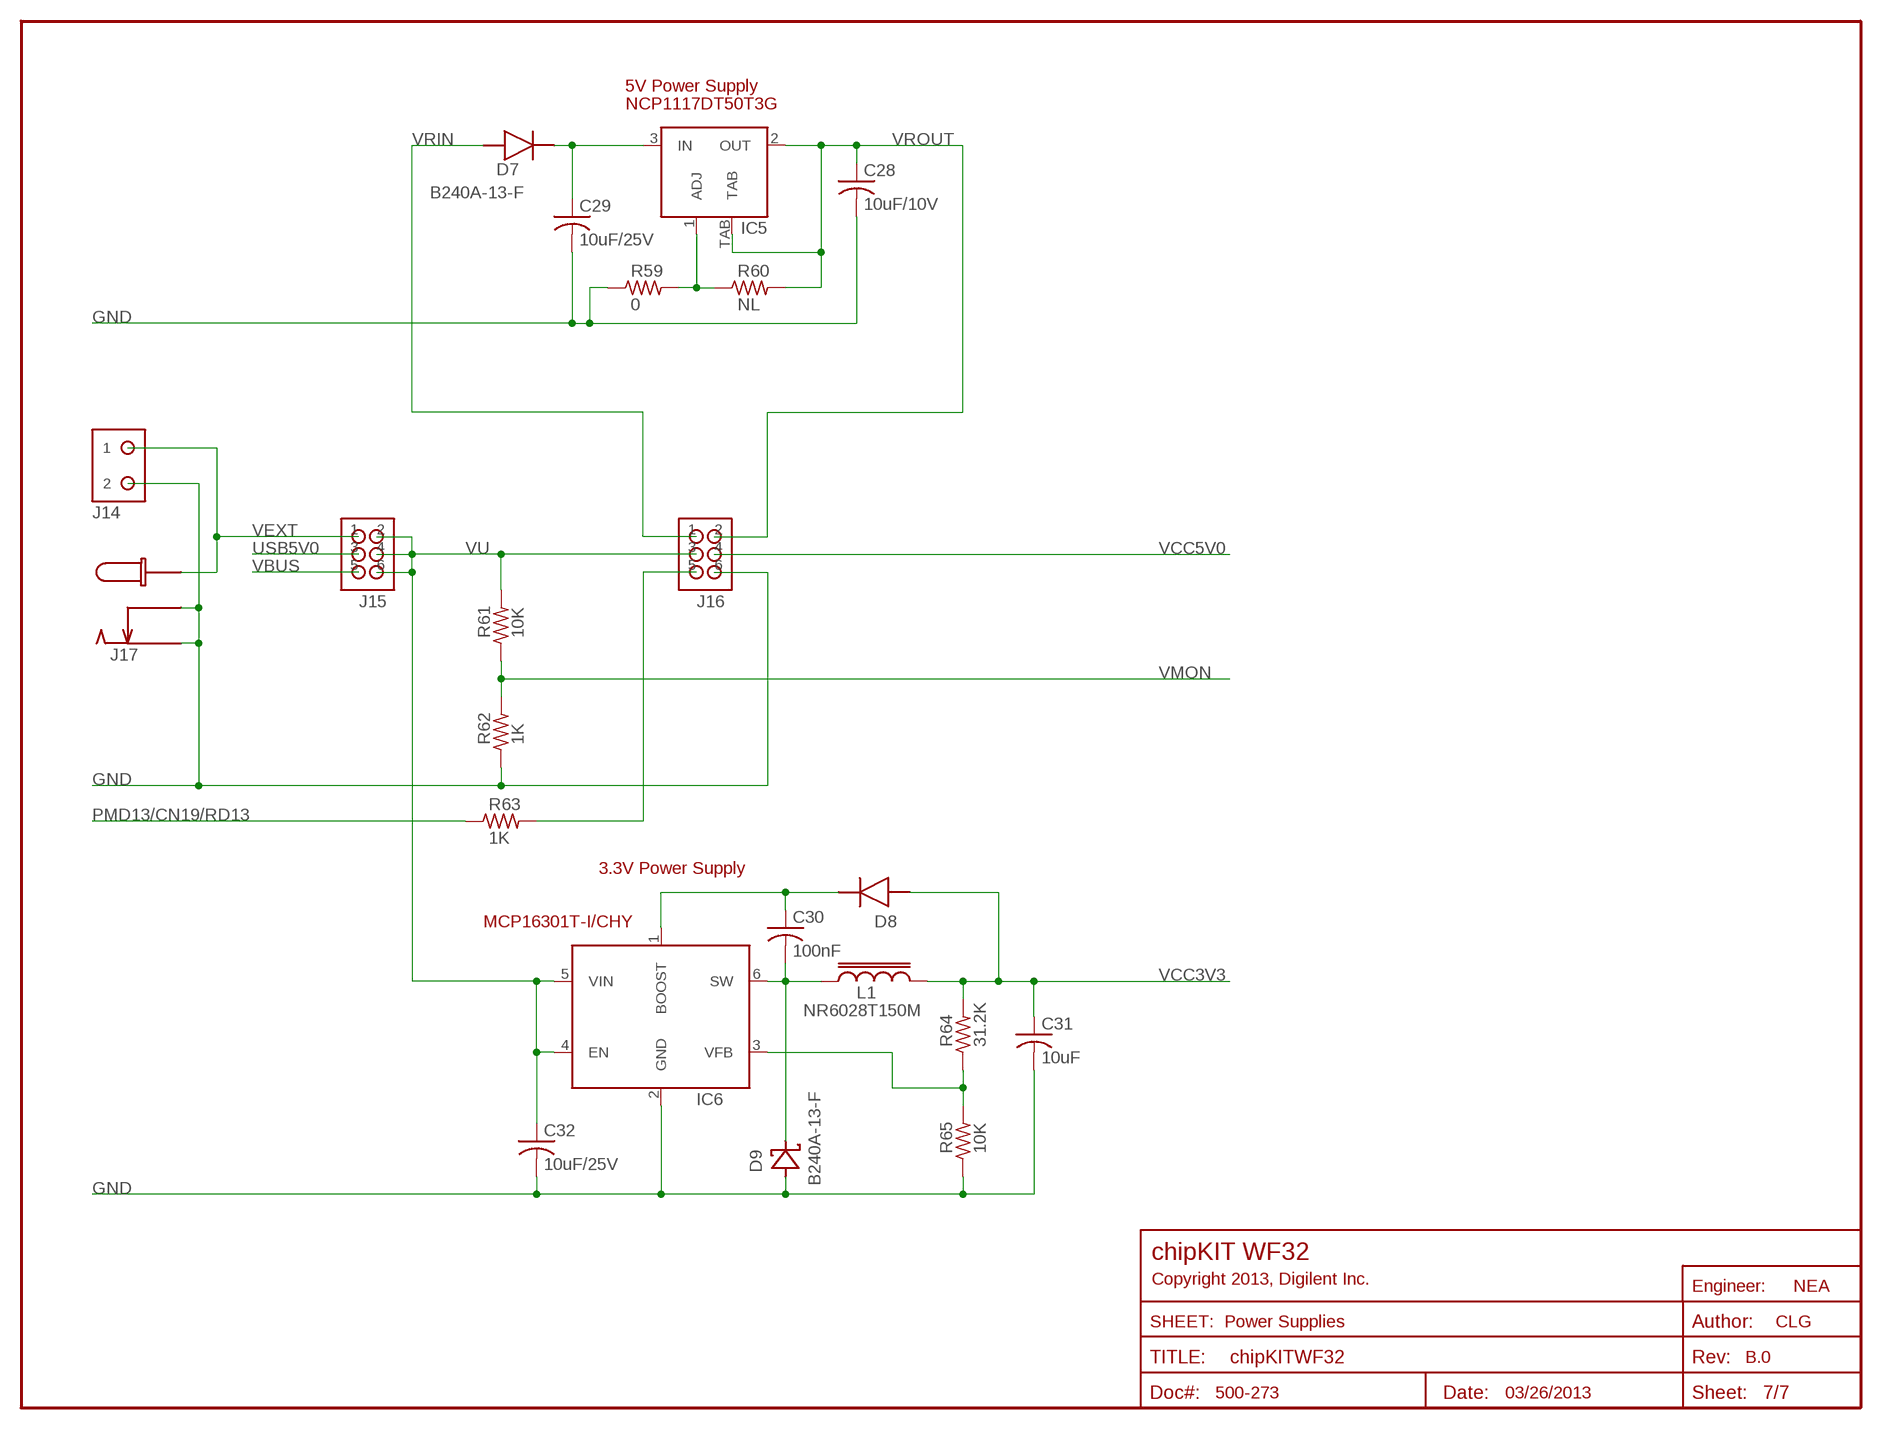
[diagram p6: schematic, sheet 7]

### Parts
C28  10uF/10V  CAP-S0805S  [C0805S]
C29  10uF/25V  CAP-S1206S  [C1206S]
C30  100nF  CAP-S0402S  [C0402S]
C31  10uF  CAP-S0805S  [C0805S]
C32  10uF/25V  CAP-S1206S  [C1206S]
D7  B240A-13-F  DIODESMA  [SMA]
D8  CDSU4148  DIODE0603S  [D0603S]
D9  B240A-13-F  SCHOTTKY-SMA  [SMA]
IC5  NCP1117DT50T3G  LM1117MP  [SOT223]
IC6  MCP16301T-I/CHY  MCP16301  [SOT23-6-CH]
J14  ST. Male  HDR-1X2  [HDR-1X2]
J15  ST. Male  JPR-2X3  [HDR-2X3]
J16  ST. Male  JPR-2X3  [HDR-2X3]
J17  CON-COAX-KLD0202-S  [KLD-0202S]
L1  NR6028T150M  IND-NR6028  [NR60XX]
R59  0  RES-S0603S  [R0603S]
R60  NL  RES-S0402S  [R0402S]
R61  10K  RES-S0402S  [R0402S]
R62  1K  RES-S0402S  [R0402S]
R63  1K  RES-S0402S  [R0402S]
R64  31.2K  RES-S0402S  [R0402S]
R65  10K  RES-S0402S  [R0402S]

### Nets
GND: C28.2 C29.2 C31.2 C32.2 D9.A IC6.2(GND) J14.2 J16.6 J17.2 J17.3 R59.1 R62.1 R65.1 ; also sheet 2,3,4,5,6
N$30: J16.5 R63.2
N$34: C30.2 D9.C IC6.6(SW) L1.1
N$35: C30.1 D8.C IC6.1(BOOST)
N$36: IC5.1(ADJ) R59.2 R60.1
N$38: IC6.3(VFB) R64.1 R65.2
N$39: C29.1 D7.C IC5.3(IN)
PMD13/CN19/RD13: R63.1 ; also sheet 5
USB5V0: J15.3 ; also sheet 2
VBUS: J15.5 ; also sheet 2,6
VCC3V3: C31.1 D8.A L1.2 R64.2 ; also sheet 2,4,6
VCC5V0: J16.4 ; also sheet 2,6
VEXT: J14.1 J15.1 J17.1 ; also sheet 2
VMON: R61.1 R62.2 ; also sheet 4
VRIN: D7.A J16.1
VROUT: C28.1 IC5.2(OUT) IC5.TAB J16.2 R60.2
VU: C32.1 IC6.4(EN) IC6.5(VIN) J15.2 J15.4 J15.6 J16.3 R61.2

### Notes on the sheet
- 5V Power Supply
- NCP1117DT50T3G
- 3.3V Power Supply
- chipKIT WF32
- Copyright 2013, Digilent Inc.
- NEA
- Power Supplies | CLG
- B.0
- 500-273 | 03/26/2013

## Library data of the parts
BTN1-BTN3 = Mechanical:SW-P8008: 153-000: SPST, Push button, momentary
C1-C32 = Discrete:CAP: Capacitor
D1 = Discrete:BAV99W: BAV99W Dual Surface Mount Switching Diode
D2 = Discrete:NSQA6V8: Low Capacitance Quad ESD Protection Array
D3-D6 = Discrete:BAV70S: High Speed Switching Diode Array
D7 D8 = Discrete:DIODE: Diode
D9 = Discrete:SCHOTTKY: Generic Schotkey diode
IC1 = IC:FT232R: FTDI USB UART Serial Converter
IC2 = Microchip:PIC32MX7X5F*L: High Performance, USB, CAN and Ethernet 32-Bit Flash Microcontroller
IC3 = Microchip:MRF24WB0MA: 2.4 GHz, IEEE Std. 802.11b RF Tranciver Module
IC4 = TI:TPS2041B: Current Limited, Power Distribution Switch
IC5 = IC:LM1117: LM1117 Adjustable voltage regulator, 1.2V dropout
IC6 = Microchip:MCP16301: Microchip MCP16301 High Voltage Input Integrated Switch Step-Down Regulator 600mA, 2 -15V Out, 4-30V In
J1 = Mechanical:USB-AB-MINI: Kycon KMAB-SMT-5S Mini USB AB type connector
J2 = Mechanical:HDR-1X4
J3 = Mechanical:HDR-1X8
J4 J5 = Mechanical:HDR-1X1
J6 J14 = Mechanical:HDR-1X2
J7 J9 = Mechanical:HDR-2X8: 100mil 2x8 header
J8 = Mechanical:HDR-2X6: 2x6 header with 42mil holes and 100mil spacing
J10 = Mechanical:HDR-2X3
J11 = Mechanical:2908-05WB-MG: 3M Card Connector microSD
J12 = Mechanical:USB-AB-MICRO
J13 = Mechanical:USB-A: Kycon KUSB-AS-1 USB Type A connector
J15 J16 = Mechanical:JPR-2X3: Jumper Block: 2x3
J17 = Mechanical:CON-COAX: COAX Power Connector
JP1 JP8 JP9 JP11 = Mechanical:JPR-1X2
JP2 = Mechanical:HDR-1X6-OFFSET: 42 mil hole pattern with 16mil offset for jtag connector
JP3-JP7 JP10 = Mechanical:JPR-1X3
L1 = Discrete:IND: Inductors
LD1-LD6 = Discrete:LED: Discrete LED
LOGO1 = Logo:DIGILENT_INC
LOGO2 = Logo:CE: European Union CE Logo
LOGO3 = Logo:CHIPKIT: Microchip chipKIT Logo
LOGO4 = Logo:WEEE: WEEE Symbol
LOGO5 = Logo:ROHS-CHINA: Chinese ROHS symbol logo
Q1 Q2 = Discrete:MBT3904DW1T1: On-Semiconductor MBT3904DW1T1 Dual General Purpose Transistors
R1-R65 = Discrete:RES: Resistor
U$1 = Logo:CHIPKIT_WF32_LOGO
VR1 = Discrete:POT
X1 X2 = Discrete:XTAL: Quartz Crystal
